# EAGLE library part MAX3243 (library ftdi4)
MAX3243 RS232 interface 5 receive lines 3 line drives 5V or 3.3V operating voltage
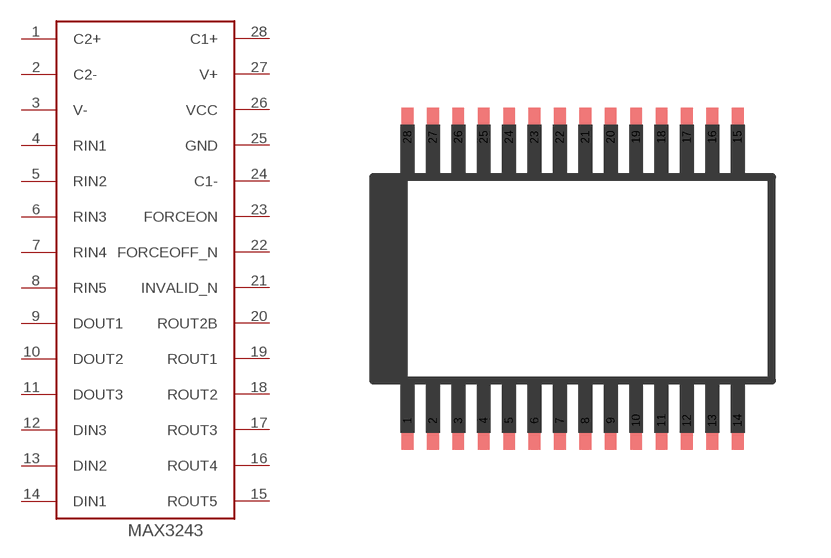
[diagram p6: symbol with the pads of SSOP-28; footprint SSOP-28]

Designator prefix -

## MAX3243  [SSOP-28]
1  C2+
2  C2-
3  V-
4  RIN1
5  RIN2
6  RIN3
7  RIN4
8  RIN5
9  DOUT1
10  DOUT2
11  DOUT3
12  DIN3
13  DIN2
14  DIN1
15  ROUT5
16  ROUT4
17  ROUT3
18  ROUT2
19  ROUT1
20  ROUT2B
21  INVALID_N
22  FORCEOFF_N
23  FORCEON
24  C1-
25  GND
26  VCC
27  V+
28  C1+

## Footprint SSOP-28 (pad centres in mm)
Shrink Small Outline Package: SSOP-28
smd 0.3 x 1.5: 1 -4.225,-3.625; 2 -3.575,-3.625; 3 -2.925,-3.625; 4 -2.275,-3.625; 5 -1.625,-3.625; 6 -0.975,-3.625; 7 -0.325,-3.625; 8 0.325,-3.625; 9 0.975,-3.625; 10 1.625,-3.625; 11 2.275,-3.625; 12 2.925,-3.625; 13 3.575,-3.625; 14 4.225,-3.625; 15 4.225,3.625; 16 3.575,3.625; 17 2.925,3.625; 18 2.275,3.625; 19 1.625,3.625; 20 0.975,3.625; 21 0.325,3.625; 22 -0.325,3.625; 23 -0.975,3.625; 24 -1.625,3.625; 25 -2.275,3.625; 26 -2.925,3.625; 27 -3.575,3.625; 28 -4.225,3.625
